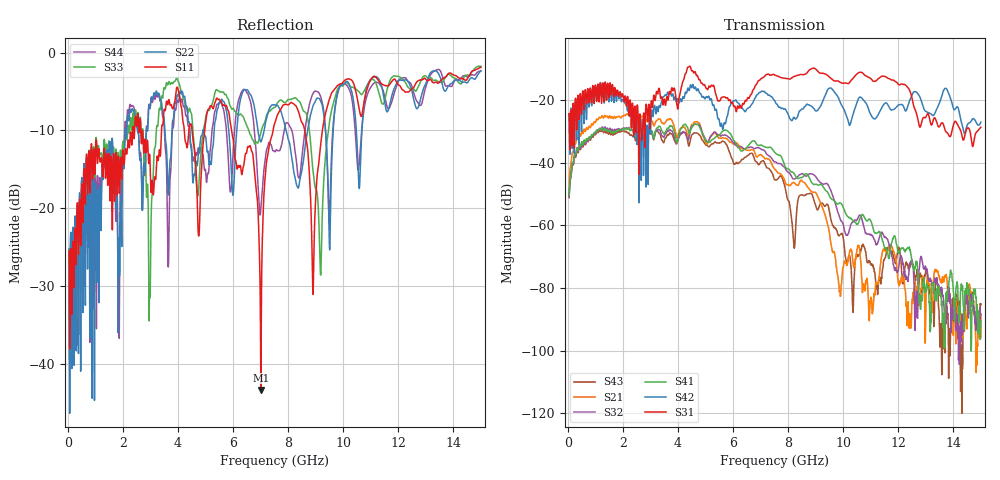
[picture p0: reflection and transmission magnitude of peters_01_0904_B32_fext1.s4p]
# MHZ S RI R 50.00
! FREQ  S11  S12  S13  S14
!  S21  S22  S23  S24
!  S31  S32  S33  S34
!  S41  S42  S43  S44
!  REAL  IMAG  REAL  IMAG  REAL  IMAG  REAL  IMAG
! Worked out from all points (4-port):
!   1496 points, 50 MHz to 15 GHz, reference 50 ohm
!   strongest paths, dB at 50 MHz, 3.79 GHz, 7.53 GHz, 11.27 GHz, 15 GHz:
!     S31: -24.4, -16.2, -12.1, -13.2, -28.7
!     S42: -24.4, -18.4, -20.5, -24.7, -27.1
!     S41: -50.4, -28.3, -36.8, -62.3, -90.4
!     S32: -50.7, -30.0, -39.7, -65.2, -88.2
!     S21: -46.9, -26.7, -42.2, -78.8, -95.8
!     S43: -51.2, -31.0, -45.5, -80.1, -85.1
!   lowest |S11| = -43.3 dB at 7.01 GHz (marker M1), VSWR 1.01, Z = 50.7 - j0.146 ohm
!   |S11| at or under -10 dB: start of sweep to 2.355 GHz; 2.654 GHz to 3.404 GHz (749.4 MHz wide, 24.7 % of centre); 5.951 GHz to 7.453 GHz (1.503 GHz wide, 22.4 % of centre)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
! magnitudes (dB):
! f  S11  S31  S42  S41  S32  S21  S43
! 50 MHz  -25.5  -24.4  -24.4  -50.4  -50.7  -46.9  -51.2
! 3.99 GHz  -4.6  -22.9  -19.6  -33.0  -33.2  -31.6  -33.0
! 7.01 GHz  -43.3  -13.3  -17.4  -34.4  -35.6  -37.4  -39.8
! 7.63 GHz  -7.9  -12.4  -21.9  -37.5  -40.3  -43.3  -45.2
! 9.18 GHz  -11.9  -11.5  -21.9  -47.0  -46.5  -52.9  -53.0
! 9.88 GHz  -4.0  -14.3  -20.5  -52.9  -57.6  -80.7  -63.1
! 15 GHz  -1.9  -28.7  -27.1  -90.4  -88.2  -95.8  -85.1
